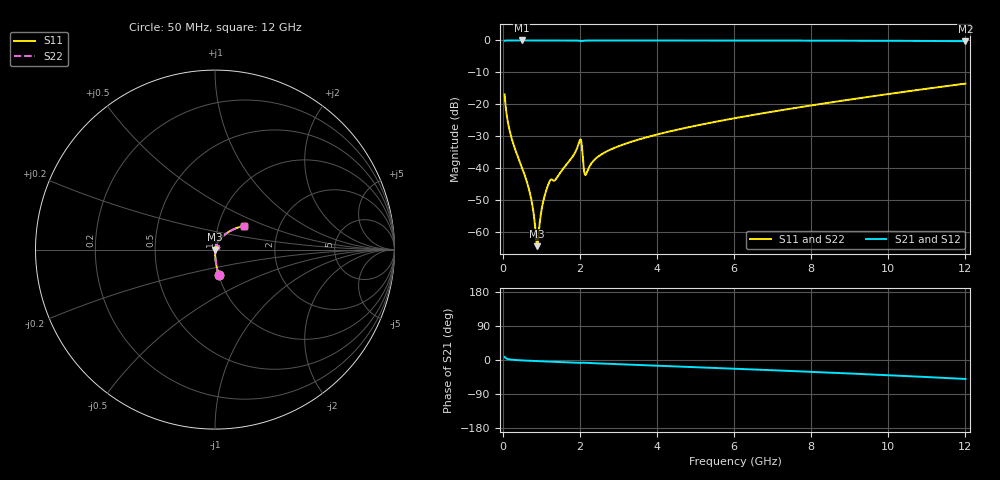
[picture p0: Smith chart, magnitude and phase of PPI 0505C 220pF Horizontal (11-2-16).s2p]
# MHz S MA R 50
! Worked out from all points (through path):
!   1601 points, 50 MHz to 12 GHz, reference 50 ohm
!   highest |S21| = 0.00 dB at 490.7 MHz (marker M1); lowest = -0.2 dB at 12 GHz (marker M2)
!   group delay of S21, straight-line fit = 11.6 ps
!   lowest |S11| = -64.6 dB at 894 MHz (marker M3), VSWR 1.00, Z = 50.1 - j0.00553 ohm
!   |S11| at or under -10 dB: start of sweep to end of sweep
!   |S22| runs from -64.6 to -13.6 dB; largest |S21 - S12| = 0
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50  0.1425 -81.9  0.9896 8.0  0.9896 8.0  0.1425 -81.9
214.3125  0.03182 -88.3  0.9991 1.1  0.9991 1.1  0.03182 -88.3
490.6562  0.01044 -88.6  0.9995 -1.0  0.9995 -1.0  0.01044 -88.6
714.7188  0.003813 -84.3  0.9994 -2.1  0.9994 -2.1  0.003813 -84.3
856.625  0.0009415 -55.4  0.9994 -2.8  0.9994 -2.8  0.0009415 -55.4
893.9688  0.0005887 -5.4  0.9994 -2.9  0.9994 -2.9  0.0005887 -5.4
931.3125  0.0009111 45.0  0.9993 -3.1  0.9993 -3.1  0.0009111 45.0
1058.281  0.003088 72.7  0.9992 -3.6  0.9992 -3.6  0.003088 72.7
1207.656  0.005959 70.8  0.9984 -4.3  0.9984 -4.3  0.005959 70.8
1401.844  0.006925 72.9  0.9984 -5.0  0.9984 -5.0  0.006925 72.9
1820.094  0.01517 76.8  0.9981 -6.8  0.9981 -6.8  0.01517 76.8
1984.406  0.02546 58.3  0.9893 -7.8  0.9893 -7.8  0.02546 58.3
2044.156  0.02446 19.1  0.9779 -7.3  0.9779 -7.3  0.02446 19.1
2118.844  0.008395 22.9  0.9926 -7.2  0.9926 -7.2  0.008395 22.9
2171.125  0.008158 54.0  0.9959 -7.5  0.9959 -7.5  0.008158 54.0
2372.781  0.01324 74.8  0.9982 -8.5  0.9982 -8.5  0.01324 74.8
2671.531  0.01776 76.5  0.9985 -9.8  0.9985 -9.8  0.01776 76.5
4038.312  0.03377 73.0  0.998 -15.1  0.998 -15.1  0.03377 73.0
6025  0.06027 65.7  0.9964 -23.0  0.9964 -23.0  0.06027 65.7
8019.156  0.09584 57.7  0.9933 -31.3  0.9933 -31.3  0.09584 57.7
10013.31  0.1445 49.0  0.9869 -40.2  0.9869 -40.2  0.1445 49.0
12000  0.2099 39.3  0.9745 -50.0  0.9745 -50.0  0.2099 39.3
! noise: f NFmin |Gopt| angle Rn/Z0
50  0.0003253  0.84  0.29  0.0004305
1372  0.004832  0.7233  4.481  0.00346
2701  0.005711  0.5788  8.684  0.002452
4031  0.007067  0.5149  12.71  0.002513
5360  0.008698  0.4882  16.65  0.002858
6682  0.01034  0.4731  20.43  0.003239
8012  0.01205  0.4655  24.09  0.00366
9341  0.01384  0.4639  27.61  0.004135
1.067e+04  0.01575  0.4674  31  0.004686
1.2e+04  0.01783  0.4756  34.28  0.005339
